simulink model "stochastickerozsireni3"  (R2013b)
settings: Solver=FixedStepDiscrete  StartTime=0.0  StopTime=132.0  FixedStep=0.1  RelTol=1e-3
libraries: simulink x6

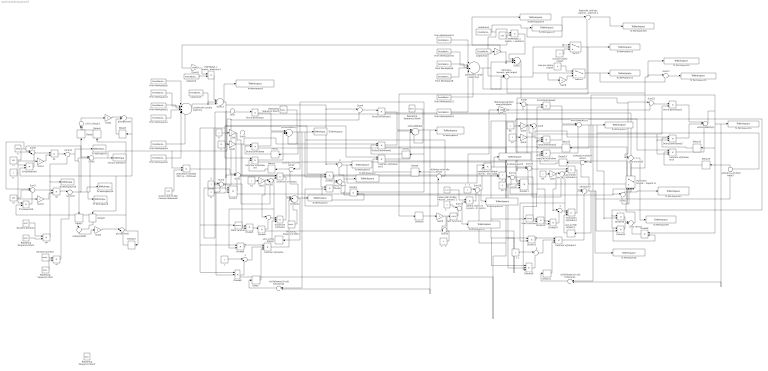
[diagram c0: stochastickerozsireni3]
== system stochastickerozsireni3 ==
  " " : Sum  Inputs=|++
  " x1(t-1) POC PODM?" : Delay  DelayLength=1  InitialCondition=0
  " x1(t-1) POC PODM?1" : Delay  DelayLength=1  InitialCondition=0
  " x(t)Followera1+x(t)Followera1" : Sum  Inputs=|++
  " x(t)Followera1+x(t)Followera2" : Sum  Inputs=|++
   x(t)Vudce+x(t)Followera{1..4} (4 alike) : Sum  Inputs=|++
  " x2t-1-x2expt-1" : Sum  Inputs=|+-
  " 1" : Sum  Inputs=|+-
  " 2" : Sum  Inputs=|++
  " 2A+2K1" : Sum  Inputs=|++
  " 2A+2K2" : Sum  Inputs=|++
  " 3" : Sum  Inputs=|+-
  " A*x1+A*xV" : Sum  Inputs=|+++
  " A*x1+A*xV1" : Sum  Inputs=|+++
  " P" : Sum  Inputs=|+-
  " prednostni vyroba elektriny" : Sum  Inputs=|++++++
  " prednostni vyroba elektriny1" : Sum  Inputs=|++++++
  " q1expectedt" : Sum  Inputs=|++
  " q1rand" : Sum  Inputs=|++
  " q1rand1" : Sum  Inputs=|++
  " q2expectedt " : Sum  Inputs=|++
  " x(t)Vudce" : Sum  Inputs=|++-+
  " x(t)Vudce1" : Sum  Inputs=|++-
  " x2expectedt1" : Sum  Inputs=|+-
  " xFOLLOWER1(t)" : Sum  Inputs=|++-+
  " xFOLLOWER1(t)1" : Sum  Inputs=|++-
  " xFOLLOWER2(t)" : Sum  Inputs=|++-+
  " xFOLLOWER2(t)1" : Sum  Inputs=|++-
  "           " : Gain
  "              " : Constant  Value=1.05
  1 : Constant
  "1 " : Constant
  "1    " : Constant
  1    1 : Constant  Value=-1
  1    2 : Constant
  1 1 : Constant
  2 : Constant
  A : Constant
  A1 : Constant
  "Cena je jednotk.N " : ToWorkspace  VariableName=Puhli  SampleTime=-1  SaveFormat=Timeseries
  Delay{,1..16} (17 alike) : Delay  DelayLength=1  InitialCondition=0
  Divide{1..2,5,7,9..10,13,15} (8 alike) : Product  Inputs=**
  Divide11 : Product  Inputs=***/
  Divide{4,6,12,14} (4 alike) : Product  Inputs=*/
  Divide16 : Product  Inputs=**/
  Divide3 : Product  Inputs=***/
  Divide8 : Product  Inputs=**/
  DruhyClenFollowa{,1..3} (4 alike) : Product  Inputs=**/
  From Workspace1 : FromWorkspace  VariableName=FVE  SampleTime=0
  From Workspace10 : FromWorkspace  VariableName=JE  SampleTime=0
  From Workspace11 : FromWorkspace  VariableName=ostatni  SampleTime=0
  From Workspace12 : FromWorkspace  VariableName=bioplyn  SampleTime=0
  From Workspace13 : FromWorkspace  VariableName=biomasa  SampleTime=0
  From Workspace2 : FromWorkspace  VariableName=VE  SampleTime=0
  From Workspace3 : FromWorkspace  VariableName=JE  SampleTime=0
  From Workspace4 : FromWorkspace  VariableName=ostatni  SampleTime=0
  From Workspace5 : FromWorkspace  VariableName=bioplyn  SampleTime=0
  From Workspace6 : FromWorkspace  VariableName=biomasa  SampleTime=0
  From Workspace8 : FromWorkspace  VariableName=FVE  SampleTime=0
  From Workspace9 : FromWorkspace  VariableName=VE  SampleTime=0
  Gain{,1..7} (8 alike) : Gain  Gain=2
  Gain10 : Gain  Gain=1.14285714286
  Gain8 : Gain  Gain=-1
  Gain9 : Gain  Gain=-1
  K : Constant  Value=15
  K1 : Constant
  K2 : Constant
  K3 : Constant
  MALEusporyprofolloweryzRozsahu : Gain  Gain=0.85
  Math Function : Math  Operator=square
  Math Function1 : Math  Operator=square
  Math Function2 : Math  SampleTime=0.1
  N : Constant  Value=3
  N1 : Constant  Value=3
  "POPTAVKA = spotreba + export - levnejsi elektrina " : Product  Inputs=**
  POPTAVKA = spotreba + export - levnejsi elektrina 1 : Product  Inputs=**
  Podminka Dostatecnych kapacit el : Switch
  Poptavka celk bez exportu - Qostatnich 1 : Sum  Inputs=|+-
  PrvniClenFollowa{,1..3} (4 alike) : Product  Inputs=*/
  Random Number : RandomNumber  Mean=1  SampleTime=0.1
  Random Number1 : RandomNumber  Mean=1  SampleTime=0.1
  Repeating Sequence Stair : simulink/Sources/Repeating Sequence Stair  OutValues="[360 0 0 0 0 0 0 0 0 0 0 0 0 0 0 0 0 0 0 0 0 0 0 0 0 0 0 0 0 0 0 0 0 0 0 0 0 0 0 0 0 0 0 0 0 0 0 0 0 0 0 0 0 0 0 0 0 0 0 0 0 0 0 0 0 0 0 0 0 0 0 0 0 0 0 0 0 0 0 0 0 0 0 0 0 0 0 0 0 0 0 0 0 0 0 0 0 0 0 0 -360 0 0 0 0 0 0 0 0 0 0 0 0 0 0 0 0 0 0 0 0 0 0 0 0 0 0 0 0 0 0 0 0 0 0 0 0 0 0 0 0 0 0 0 0 0 0 0 0 0 0 0 0 0 0 0 0 0 0 0 0 0 0 0 0 0 0 0 0 0 0 0 0 0 0 0 0 0 0 0 0 0 0 0 0 0 0 0 0 0 0 0 0 0 0 0 0 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"  tsamp=-1  OutMin=[]  OutMax=[]  OutDataTypeStr=double  OutputDataTypeScalingMode=double  OutDataType=fixdt(0,8)  ConRadixGroup=Best Precision: Vector-wise  OutScaling=2^-12
  Repeating Sequence Stair1 : simulink/Sources/Repeating Sequence Stair  OutValues="[360 0 0 0 0 0 0 0 0 0 0 0 0 0 0 0 0 0 0 0 0 0 0 0 0 0 0 0 0 0 0 0 0 0 0 0 0 0 0 0 0 0 0 0 0 0 0 0 0 0 0 0 0 0 0 0 0 0 0 0 0 0 0 0 0 0 0 0 0 0 0 0 0 0 0 0 0 0 0 0 0 0 0 0 0 0 0 0 0 0 0 0 0 0 0 0 0 0 0 0 -360 0 0 0 0 0 0 0 0 0 0 0 0 0 0 0 0 0 0 0 0 0 0 0 0 0 0 0 0 0 0 0 0 0 0 0 0 0 0 0 0 0 0 0 0 0 0 0 0 0 0 0 0 0 0 0 0 0 0 0 0 0 0 0 0 0 0 0 0 0 0 0 0 0 0 0 0 0 0 0 0 0 0 0 0 0 0 0 0 0 0 0 0 0 0 0 0 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"  tsamp=-1  OutMin=[]  OutMax=[]  OutDataTypeStr=double  OutputDataTypeScalingMode=double  OutDataType=fixdt(0,8)  ConRadixGroup=Best Precision: Vector-wise  OutScaling=2^-12
  Repeating Sequence Stair{2,4..6} (4 alike) : simulink/Sources/Repeating Sequence Stair  OutValues="[180 0 0 0 0 0 0 0 0 0 0 0 0 0 0 0 0 0 0 0 0 0 0 0 0 0 0 0 0 0 0 0 0 0 0 0 0 0 0 0 0 0 0 0 0 0 0 0 0 0 0 0 0 0 0 0 0 0 0 0 0 0 0 0 0 0 0 0 0 0 0 0 0 0 0 0 0 0 0 0 0 0 0 0 0 0 0 0 0 0 0 0 0 0 0 0 0 0 0 0 -180 0 0 0 0 0 0 0 0 0 0 0 0 0 0 0 0 0 0 0 0 0 0 0 0 0 0 0 0 0 0 0 0 0 0 0 0 0 0 0 0 0 0 0 0 0 0 0 0 0 0 0 0 0 0 0 0 0 0 0 0 0 0 0 0 0 0 0 0 0 0 0 0 0 0 0 0 0 0 0 0 0 0 0 0 0 0 0 0 0 0 0 0 0 0 0 0 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"  tsamp=-1  OutMin=[]  OutMax=[]  OutDataTypeStr=double  OutputDataTypeScalingMode=double  OutDataType=fixdt(0,8)  ConRadixGroup=Best Precision: Vector-wise  OutScaling=2^-12
  "Spotreba - levnejsiEl - Qvyr (esi deficit elektriny doma, pak Import" : Sum  Inputs=|+--
  Sum{,4,8,12,14,17..19} (8 alike) : Sum  Inputs=|+-
  Sum1 : Sum  Inputs=|++
  Sum10 : Sum  Inputs=|-+-
  Sum11 : Sum  Inputs=|-+
  Sum13 : Sum  Inputs=|++-
  Sum15 : Sum  Inputs=|++-
  Sum16 : Sum  Inputs=|++
  Sum2 : Sum  Inputs=|-+-
  Sum3 : Sum  Inputs=|-+
  Sum5 : Sum  Inputs=|+--
  Sum6 : Sum  Inputs=|+--
  Sum7 : Sum  Inputs=|+--
  Sum9 : Sum  Inputs=|++
  Switch : Switch
  Switch1 : Switch
  To Workspace : ToWorkspace  VariableName=qFolloweraVyrobceUhli1  SampleTime=-1  SaveFormat=Timeseries
  To Workspace1 : ToWorkspace  VariableName=qVudceVyrobceUhli  SampleTime=-1  SaveFormat=Timeseries
  To Workspace10 : ToWorkspace  VariableName=qFolloweraObchodnika2  SampleTime=-1  SaveFormat=Timeseries
  To Workspace11 : ToWorkspace  VariableName=KoefRedukceNakladuZimportu  SampleTime=-1  SaveFormat=Timeseries
  To Workspace12 : ToWorkspace  VariableName=qExportovane  SampleTime=-1  SaveFormat=Timeseries
  To Workspace13 : ToWorkspace  VariableName=qImportovane  SampleTime=-1  SaveFormat=Timeseries
  To Workspace14 : ToWorkspace  VariableName=RedukceNakladuCelkemUvudce  SampleTime=-1  SaveFormat=Timeseries
  To Workspace15 : ToWorkspace  VariableName=qCelkObchMinusExportovane  SampleTime=-1  SaveFormat=Timeseries
  To Workspace16 : ToWorkspace  VariableName=qCelkObc  SampleTime=-1  SaveFormat=Timeseries
  To Workspace17 : ToWorkspace  VariableName=POPTAVKACELKEM  SampleTime=-1  SaveFormat=Timeseries
  To Workspace18 : ToWorkspace  VariableName=EXPORTREAL  SampleTime=-1  SaveFormat=Timeseries
  To Workspace19 : ToWorkspace  VariableName=wazcher  SampleTime=-1  SaveFormat=Timeseries
  To Workspace2 : ToWorkspace  VariableName=PelektrinyZuhli  SampleTime=-1  SaveFormat=Timeseries
  To Workspace20 : ToWorkspace  VariableName=NETPOPTAVKA  SampleTime=-1  SaveFormat=Timeseries
  To Workspace21 : ToWorkspace  VariableName=NeniKapacita  SampleTime=-1  SaveFormat=Timeseries
  To Workspace22 : ToWorkspace  VariableName=qCelkVyr  SampleTime=-1  SaveFormat=Timeseries
  To Workspace23 : ToWorkspace  VariableName=NakladyVudceCelkemPoRedukci  SampleTime=-1  SaveFormat=Timeseries
  To Workspace24 : ToWorkspace  VariableName=wazcher1  SampleTime=-1  SaveFormat=Timeseries
  To Workspace3 : ToWorkspace  VariableName=qFolloweraVyrobceUhli2  SampleTime=-1  SaveFormat=Timeseries
  To Workspace4 : ToWorkspace  VariableName=poptavkaUvyrobcuElzUhli  SampleTime=-1  SaveFormat=Timeseries
  To Workspace5 : ToWorkspace  VariableName=q1uhli  SampleTime=-1  SaveFormat=Timeseries
  To Workspace6 : ToWorkspace  VariableName=q2uhli  SampleTime=-1  SaveFormat=Timeseries
  To Workspace7 : ToWorkspace  VariableName=qFolloweraObchodnika1  SampleTime=-1  SaveFormat=Timeseries
  To Workspace8 : ToWorkspace  VariableName=qVudceObchodnika  SampleTime=-1  SaveFormat=Timeseries
  To Workspace9 : ToWorkspace  VariableName=PmaloobchodniObchodniku  SampleTime=-1  SaveFormat=Timeseries
  "a " : Constant  Value=6000
  "b " : Constant
  b*q1expected : Product
  b*q2expected : Product
  beta1 : Gain
  beta2 : Gain
  c1 : Constant  Value=400
  c2 : Constant  Value=400
  druhyClen x(t)Vudce : Product  Inputs=*/*
  druhyClen x(t)Vudce1 : Product  Inputs=*/*
  "jednotkove naklady ČEZ obchodníka který má mít dominant.pozici 44% trzni podil " : Product  Inputs=**
  jednotkove naklady ČEZ výrobce P-Pinhouse : Product  Inputs=**
  nula pro zadny export : Constant  Value=0
  nula pro zadny import : Constant  Value=0
  p=b-a*sumaQ : Sum  Inputs=|+-
  poptavka : FromWorkspace  VariableName=nettospotreba  SampleTime=0
  poptavka1 : FromWorkspace  VariableName=nettospotreba  SampleTime=0
  poptavka2 : FromWorkspace  VariableName=vyvoz  SampleTime=0
  poptavka3 : FromWorkspace  VariableName=vyvoz  SampleTime=0
  prvniClen x(t)Vudce : Product  Inputs=*/
  prvniClen x(t)Vudce1 : Product  Inputs=*/
  q1 : Product  Inputs=*/
  q2 : Product  Inputs=*/
  q3 : Product  Inputs=**
  q4 : Product  Inputs=**
  snizeni jedn N diky inhouse dodavkam : Constant  Value=0.25
  snizeni jedn N diky inhouse dodavkam1 1 : Constant  Value=0.27
  tretiClen x(t)Followera{,1..3} (4 alike) : Product  Inputs=**/
  tretiClen x(t)Vudce : Product  Inputs=***
  tretiClen x(t)Vudce1 : Product  Inputs=***
  "zpetna vazba na zvyseni nakladu kvuli importu " : Product  Inputs=*/
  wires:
  Sum13/1 -> To Workspace4/1, Sum2/2, Sum/1, Sum4/1, " P"/1
  Sum/1 -> Divide3/1, PrvniClenFollowa/1
  Gain/1 -> " 2A+2K1"/2, Sum1/1
  K/1 -> Gain1/1
  PrvniClenFollowa/1 -> " xFOLLOWER1(t)"/1
  DruhyClenFollowa/1 -> " xFOLLOWER1(t)"/2
  tretiClen x(t)Followera/1 -> " xFOLLOWER1(t)"/3
  N/1 -> Sum3/2, Divide8/2
  1/1 -> Sum3/1
  Sum3/1 -> Divide5/1, Divide3/2
  Divide3/1 -> Sum2/3
  Sum2/1 -> prvniClen x(t)Vudce/1
  K1/1 -> Gain2/1
  Gain2/1 -> " "/1, " 2A+2K1"/1
  " 2A+2K1"/1 -> prvniClen x(t)Vudce/2, Divide4/2, druhyClen x(t)Vudce/2
  " "/1 -> druhyClen x(t)Vudce/1
  Math Function/1 -> Divide5/2
  Divide6/1 -> " "/2
  Divide5/1 -> Divide6/1
  "1 "/1 -> " 1"/1
  Divide4/1 -> tretiClen x(t)Vudce/1
  " 1"/1 -> tretiClen x(t)Vudce/2
  Divide8/1 -> " 1"/2
  Delay/1 -> tretiClen x(t)Vudce/3
  prvniClen x(t)Vudce/1 -> " x(t)Vudce"/1
  druhyClen x(t)Vudce/1 -> " x(t)Vudce"/2
  tretiClen x(t)Vudce/1 -> " x(t)Vudce"/3
  " x(t)Vudce"/1 -> " x(t)Vudce+x(t)Followera2"/2, " x(t)Vudce+x(t)Followera1"/1, Divide7/2, To Workspace1/1, " x1(t-1) POC PODM?"/1
  " x1(t-1) POC PODM?"/1 -> druhyClen x(t)Vudce/3
  Divide2/1 -> " A*x1+A*xV"/1
  Divide7/1 -> " A*x1+A*xV"/2
  Sum4/1 -> PrvniClenFollowa1/1
  Gain1/1 -> DruhyClenFollowa1/1, DruhyClenFollowa/1, Sum1/2
  A/1 -> tretiClen x(t)Followera1/1, Divide1/2, Divide7/1, Divide2/1, Divide8/1, Divide4/1, Math Function/1, Divide3/3, tretiClen x(t)Followera/1, Gain/1
  Sum1/1 -> tretiClen x(t)Followera1/3, DruhyClenFollowa1/3, PrvniClenFollowa1/2, Divide8/3, Divide3/4, Divide6/2, tretiClen x(t)Followera/3, DruhyClenFollowa/3, PrvniClenFollowa/2
  PrvniClenFollowa1/1 -> " xFOLLOWER2(t)"/1
  DruhyClenFollowa1/1 -> " xFOLLOWER2(t)"/2
  tretiClen x(t)Followera1/1 -> " xFOLLOWER2(t)"/3
  " xFOLLOWER2(t)"/1 -> " x(t)Vudce+x(t)Followera2"/1, Delay2/1, Divide1/1, To Workspace3/1, " x(t)Followera1+x(t)Followera2"/2
  " x(t)Followera1+x(t)Followera2"/1 -> Delay/1
  Divide1/1 -> " A*x1+A*xV"/3
  " xFOLLOWER1(t)"/1 -> Delay1/1, Divide2/2, " x(t)Vudce+x(t)Followera1"/2, To Workspace/1, " x(t)Followera1+x(t)Followera2"/1
  Delay1/1 -> DruhyClenFollowa/2
  Delay2/1 -> DruhyClenFollowa1/2
  " x(t)Vudce+x(t)Followera2"/1 -> Delay3/1
  Delay3/1 -> tretiClen x(t)Followera/2
  " x(t)Vudce+x(t)Followera1"/1 -> Delay4/1
  Delay4/1 -> tretiClen x(t)Followera1/2
  "a "/1 -> Sum7/1, Sum5/1, Sum6/1
  c1/1 -> Sum6/2
  "b "/1 -> Gain4/1, b*q1expected/1, Gain3/1, b*q2expected/1
  b*q2expected/1 -> Sum6/3
  Sum6/1 -> q1/1
  Gain3/1 -> q1/2
  c2/1 -> Sum7/2
  b*q1expected/1 -> Sum7/3
  Sum7/1 -> q2/1
  Gain4/1 -> q2/2
  " q2expectedt "/1 -> Delay9/1, Delay8/1, b*q2expected/2
  " x2expectedt1"/1 -> beta2/1
  " x2t-1-x2expt-1"/1 -> beta1/1
  Delay5/1 -> " x2t-1-x2expt-1"/1
  " q1expectedt"/1 -> Delay10/1, b*q1expected/2, Delay6/1
  Delay6/1 -> " x2t-1-x2expt-1"/2
  beta1/1 -> " q2expectedt "/1
  Delay7/1 -> " x2expectedt1"/1
  Delay8/1 -> " x2expectedt1"/2
  beta2/1 -> " q1expectedt"/1
  Delay9/1 -> " q2expectedt "/2
  Delay10/1 -> " q1expectedt"/2
  Sum15/1 -> Sum10/2, Sum8/1, Sum12/1, p=b-a*sumaQ/1
  Sum8/1 -> Divide11/1, PrvniClenFollowa2/1
  Gain5/1 -> " 2A+2K2"/2, Sum9/1
  K2/1 -> Gain6/1
  PrvniClenFollowa2/1 -> " xFOLLOWER1(t)1"/1
  DruhyClenFollowa2/1 -> " xFOLLOWER1(t)1"/2
  tretiClen x(t)Followera2/1 -> " xFOLLOWER1(t)1"/3
  N1/1 -> Sum11/2, Divide16/2
  2/1 -> Sum11/1
  Sum11/1 -> Divide13/1, Divide11/2
  Divide11/1 -> Sum10/3
  Sum10/1 -> prvniClen x(t)Vudce1/1
  K3/1 -> Gain7/1
  Gain7/1 -> " 2"/1, " 2A+2K2"/1
  " 2A+2K2"/1 -> prvniClen x(t)Vudce1/2, Divide12/2, druhyClen x(t)Vudce1/2
  " 2"/1 -> druhyClen x(t)Vudce1/1
  Math Function1/1 -> Divide13/2
  Divide14/1 -> " 2"/2
  Divide13/1 -> Divide14/1
  1 1/1 -> " 3"/1
  Divide12/1 -> tretiClen x(t)Vudce1/1
  " 3"/1 -> tretiClen x(t)Vudce1/2
  Divide16/1 -> " 3"/2
  Delay11/1 -> tretiClen x(t)Vudce1/3
  prvniClen x(t)Vudce1/1 -> " x(t)Vudce1"/1
  druhyClen x(t)Vudce1/1 -> " x(t)Vudce1"/2
  tretiClen x(t)Vudce1/1 -> " x(t)Vudce1"/3
  " x(t)Vudce1"/1 -> " x(t)Vudce+x(t)Followera4"/2, " x(t)Vudce+x(t)Followera3"/1, Divide15/2, To Workspace8/1, " x1(t-1) POC PODM?1"/1
  " x1(t-1) POC PODM?1"/1 -> druhyClen x(t)Vudce1/3
  Divide10/1 -> " A*x1+A*xV1"/1
  Divide15/1 -> " A*x1+A*xV1"/2
  p=b-a*sumaQ/1 -> To Workspace9/1
  Sum12/1 -> PrvniClenFollowa3/1
  Gain6/1 -> DruhyClenFollowa3/1, DruhyClenFollowa2/1, Sum9/2
  A1/1 -> tretiClen x(t)Followera3/1, Divide9/2, Divide15/1, Divide10/1, Divide16/1, Divide12/1, Math Function1/1, Divide11/3, tretiClen x(t)Followera2/1, Gain5/1
  Sum9/1 -> tretiClen x(t)Followera3/3, DruhyClenFollowa3/3, PrvniClenFollowa3/2, Divide16/3, Divide11/4, Divide14/2, tretiClen x(t)Followera2/3, DruhyClenFollowa2/3, PrvniClenFollowa2/2
  PrvniClenFollowa3/1 -> " xFOLLOWER2(t)1"/1
  DruhyClenFollowa3/1 -> " xFOLLOWER2(t)1"/2
  tretiClen x(t)Followera3/1 -> " xFOLLOWER2(t)1"/3
  " xFOLLOWER2(t)1"/1 -> Delay13/1, Divide9/1, To Workspace10/1, " x(t)Followera1+x(t)Followera1"/2, " x(t)Vudce+x(t)Followera4"/1
  " x(t)Followera1+x(t)Followera1"/1 -> Delay11/1
  Divide9/1 -> " A*x1+A*xV1"/3
  " xFOLLOWER1(t)1"/1 -> Delay12/1, Divide10/2, " x(t)Vudce+x(t)Followera3"/2, To Workspace7/1, " x(t)Followera1+x(t)Followera1"/1
  Delay12/1 -> DruhyClenFollowa2/2
  Delay13/1 -> DruhyClenFollowa3/2
  " x(t)Vudce+x(t)Followera4"/1 -> Delay14/1
  Delay14/1 -> tretiClen x(t)Followera2/2
  " x(t)Vudce+x(t)Followera3"/1 -> Delay15/1
  Delay15/1 -> tretiClen x(t)Followera3/2
  snizeni jedn N diky inhouse dodavkam/1 -> jednotkove naklady ČEZ výrobce P-Pinhouse/2
  From Workspace5/1 -> " prednostni vyroba elektriny"/1
  From Workspace3/1 -> " prednostni vyroba elektriny"/2
  From Workspace2/1 -> " prednostni vyroba elektriny"/3
  Sum5/1 -> jednotkove naklady ČEZ výrobce P-Pinhouse/1, Sum4/2, Sum/2, "Cena je jednotk.N "/1
  From Workspace1/1 -> " prednostni vyroba elektriny"/4
  From Workspace4/1 -> " prednostni vyroba elektriny"/6
  POPTAVKA = spotreba + export - levnejsi elektrina 1/1 -> Sum13/1
  " prednostni vyroba elektriny"/1 -> Sum13/3
  From Workspace12/1 -> " prednostni vyroba elektriny1"/1
  From Workspace10/1 -> " prednostni vyroba elektriny1"/2
  From Workspace9/1 -> " prednostni vyroba elektriny1"/3
  From Workspace8/1 -> " prednostni vyroba elektriny1"/4
  From Workspace11/1 -> " prednostni vyroba elektriny1"/6
  From Workspace13/1 -> " prednostni vyroba elektriny1"/5
  poptavka1/1 -> Poptavka celk bez exportu - Qostatnich 1/1, To Workspace17/1, "POPTAVKA = spotreba + export - levnejsi elektrina "/1, "Spotreba - levnejsiEl - Qvyr (esi deficit elektriny doma, pak Import"/1
  "POPTAVKA = spotreba + export - levnejsi elektrina "/1 -> Sum15/1
  jednotkove naklady ČEZ výrobce P-Pinhouse/1 -> Sum2/1
  " P"/1 -> "jednotkove naklady ČEZ obchodníka který má mít dominant.pozici 44% trzni podil "/1, MALEusporyprofolloweryzRozsahu/1, To Workspace2/1
  "jednotkove naklady ČEZ obchodníka který má mít dominant.pozici 44% trzni podil "/1 -> To Workspace23/1, Sum10/1
  " prednostni vyroba elektriny1"/1 -> Poptavka celk bez exportu - Qostatnich 1/2, "Spotreba - levnejsiEl - Qvyr (esi deficit elektriny doma, pak Import"/2, Sum15/3
  poptavka3/1 -> Sum13/2
  nula pro zadny import/1 -> Switch/3
  Switch/1 -> Delay16/1, To Workspace13/1
  "Spotreba - levnejsiEl - Qvyr (esi deficit elektriny doma, pak Import"/1 -> Gain8/1, Switch1/2, Switch/1, Switch/2
  Switch1/1 -> Sum17/2, To Workspace12/1
  nula pro zadny export/1 -> Switch1/1
  Gain8/1 -> Switch1/3
  "           "/1 -> To Workspace18/1, Sum15/2
  poptavka2/1 -> "           "/1
  snizeni jedn N diky inhouse dodavkam1 1/1 -> "zpetna vazba na zvyseni nakladu kvuli importu "/1
  Math Function2/1 -> Sum14/2
  "1    "/1 -> Sum14/1
  Sum14/1 -> To Workspace11/1, "zpetna vazba na zvyseni nakladu kvuli importu "/2
  Gain9/1 -> Sum16/1
  1    1/1 -> Sum16/2
  Sum16/1 -> Math Function2/1
  Delay16/1 -> Gain9/1
  Sum17/1 -> To Workspace15/1
  Poptavka celk bez exportu - Qostatnich 1/1 -> To Workspace20/1
  From Workspace6/1 -> " prednostni vyroba elektriny"/5
  MALEusporyprofolloweryzRozsahu/1 -> Sum12/2, Sum8/2
  " A*x1+A*xV"/1 -> To Workspace22/1, " P"/2, Podminka Dostatecnych kapacit el/3, Sum18/1
  " A*x1+A*xV1"/1 -> Sum18/2, Podminka Dostatecnych kapacit el/1
  Sum18/1 -> To Workspace21/1, Podminka Dostatecnych kapacit el/2
  Podminka Dostatecnych kapacit el/1 -> "Spotreba - levnejsiEl - Qvyr (esi deficit elektriny doma, pak Import"/3, To Workspace16/1, Sum17/1, p=b-a*sumaQ/2
  "              "/1 -> "POPTAVKA = spotreba + export - levnejsi elektrina "/2, Gain10/1
  poptavka/1 -> POPTAVKA = spotreba + export - levnejsi elektrina 1/2
  Gain10/1 -> POPTAVKA = spotreba + export - levnejsi elektrina 1/1
  1    2/1 -> Sum19/1
  Sum19/1 -> To Workspace14/1, "jednotkove naklady ČEZ obchodníka který má mít dominant.pozici 44% trzni podil "/2
  "zpetna vazba na zvyseni nakladu kvuli importu "/1 -> Sum19/2
  " q1rand"/1 -> Delay7/1, Sum5/2, To Workspace5/1
  q1/1 -> " q1rand"/1
  " q1rand1"/1 -> To Workspace24/1, To Workspace6/1, Sum5/3, Delay5/1
  q2/1 -> " q1rand1"/1
  Repeating Sequence Stair5/1 -> " xFOLLOWER1(t)"/4
  Repeating Sequence Stair6/1 -> " xFOLLOWER2(t)"/4
  Repeating Sequence Stair4/1 -> " x(t)Vudce"/4
  Repeating Sequence Stair/1 -> q3/2
  Random Number/1 -> q3/1
  q3/1 -> " q1rand1"/2
  Repeating Sequence Stair1/1 -> q4/2
  Random Number1/1 -> q4/1
  q4/1 -> To Workspace19/1, " q1rand"/2
